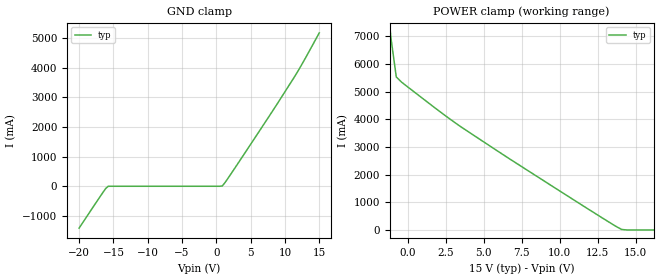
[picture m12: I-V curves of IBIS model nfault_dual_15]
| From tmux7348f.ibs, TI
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| nfault_dual_15
[Model]   nfault_dual_15
Model_type   Input
Vinl = 0.8
Vinh = 1.3
|   typ   min   max
C_comp   NA   NA
[Voltage Range]   15   NA   NA
[Temperature Range]   27   NA   NA
[Power Clamp Reference]   15   NA   NA
[GND Clamp Reference]   0   NA   NA
[GND Clamp]
|   Voltage   I(typ)   I(min)   I(max)
-20V      -1.413A    NA         NA
-16.46V   -188.9mA   NA         NA
-16.11V   -74.1mA    NA         NA
-15.76V   -925.7uA   NA         NA
858.6mV   8.913mA    NA         NA
1.566V    222.8mA    NA         NA
4.394V    1.202A     NA         NA
11.46V    3.718A     NA         NA
12.88V    4.279A     NA         NA
15V       5.173A     NA         NA
[POWER Clamp]
|   Voltage   I(typ)   I(min)   I(max)
-5V       33.27A     NA         NA
-1.465V   8.901A     NA         NA
-1.111V   6.954A     NA         NA
-757.6mV  5.534A     NA         NA
-404mV    5.345A     NA         NA
3.485V    3.736A     NA         NA
9.495V    1.591A     NA         NA
14.09V    18.22mA    NA         NA
30V       -9.981uA   NA         NA
